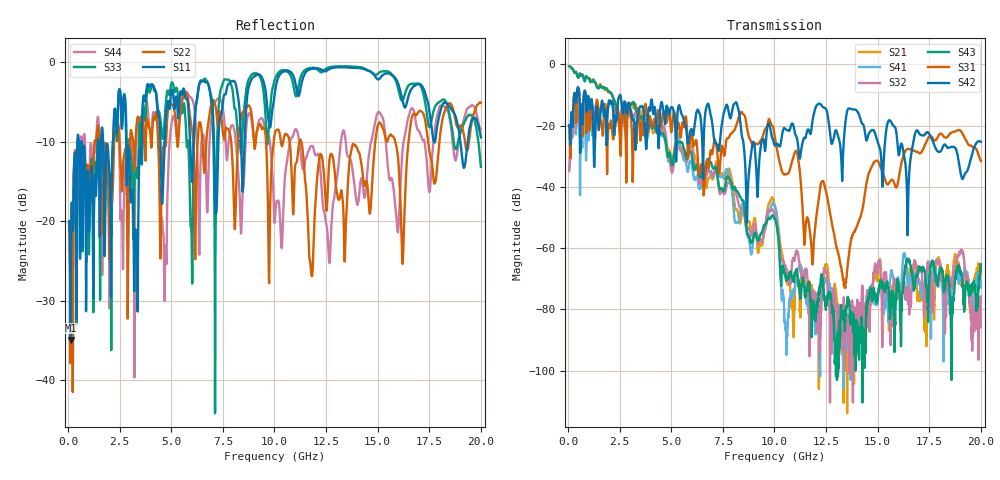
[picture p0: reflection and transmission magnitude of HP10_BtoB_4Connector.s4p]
# MHz S MA R 50.00
! FREQ  S11  S12  S13  S14
!  S21  S22  S23  S24
!  S31  S32  S33  S34
!  S41  S42  S43  S44
!  MAG  ANG  MAG  ANG  MAG  ANG  MAG  ANG
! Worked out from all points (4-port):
!   1996 points, 50 MHz to 20 GHz, reference 50 ohm
!   strongest paths, dB at 50 MHz, 5.04 GHz, 10.03 GHz, 15.02 GHz, 20 GHz:
!     S42: -19.9, -14.0, -26.6, -25.7, -25.3
!     S31: -20.0, -20.4, -24.4, -31.7, -31.6
!     S43: -0.6, -33.0, -50.7, -74.6, -65.3
!     S32: -34.7, -35.4, -49.8, -65.2, -75.8
!     S41: -34.8, -32.2, -46.8, -75.8, -72.9
!     S21: -0.6, -33.3, -46.5, -68.4, -68.8
!   lowest |S11| = -34.9 dB at 120 MHz (marker M1), VSWR 1.04, Z = 51.8 - j0.0202 ohm
!   |S11| at or under -10 dB: 645.7 MHz to 1.441 GHz (795.2 MHz wide, 76.2 % of centre); 1.697 GHz to 2.166 GHz (468.7 MHz wide, 24.3 % of centre); 2.814 GHz to 3.559 GHz (744.3 MHz wide, 23.4 % of centre)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
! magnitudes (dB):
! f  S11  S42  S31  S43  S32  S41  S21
! 50 MHz  -20.1  -19.9  -20.0  -0.6  -34.7  -34.8  -0.6
! 120 MHz  -34.9  -23.6  -26.1  -0.9  -26.9  -26.8  -0.9
! 9.77 GHz  -8.1  -20.2  -18.3  -50.4  -47.9  -47.9  -44.9
! 10.54 GHz  -1.1  -21.2  -35.9  -69.8  -66.5  -86.9  -68.8
! 13.4 GHz  -0.6  -21.4  -72.3  -81.7  -82.6  -90.8  -94.9
! 14.88 GHz  -1.8  -22.7  -31.7  -76.2  -65.1  -78.3  -67.1
! 20 GHz  -9.4  -25.3  -31.6  -65.3  -75.8  -72.9  -68.8
